(* Logix 5000 AddOnInstructionDefinition export B256_LtoE; software revision 30.00 *)

ADD_ON_INSTRUCTION D_SHR   (* revision 1.0, vendor Ken Fischer, NSWCPD, C512 *)
// DINT bit shift right of the 32-bit argument Inp_A by Inp_B bits with paddding by zeros on the right
// Revision note:
// Rev1.0: TBD - Initial Release
VAR_IN_OUT
   Inp_A : DINT; {required}   // 64-bit Integer to be right circular rotated
END_VAR
VAR_INPUT
   Inp_B : INT; {required}   // Number of bits to shift
END_VAR
VAR_IN_OUT
   Out : DINT; {required}   // Result
END_VAR
VAR
   BSR_Cntrl : CONTROL := (LEN := 32);
   ONS : BOOL;
   Source_Bit : BOOL;
   Wrk_InpA : DINT[2];
END_VAR

ROUTINE Logic   (* ladder *)
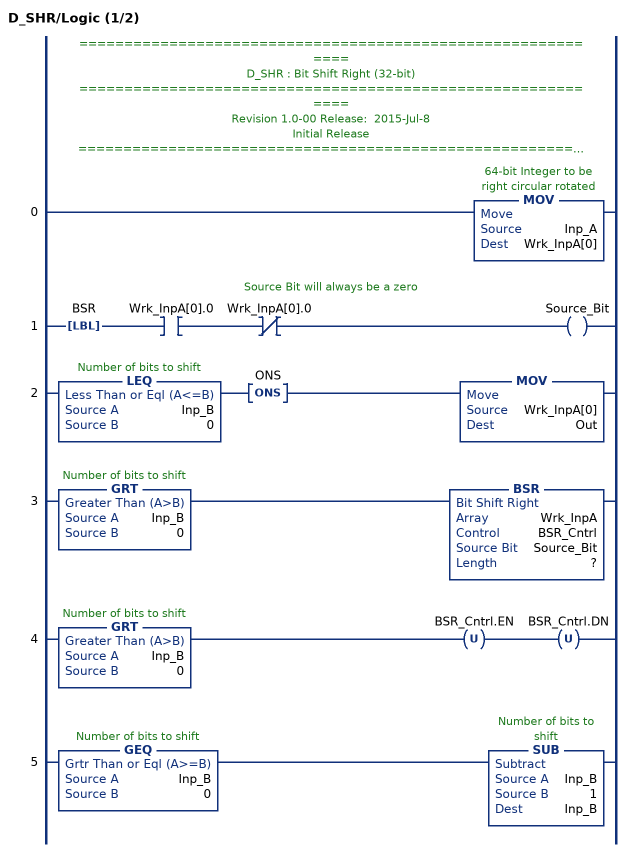
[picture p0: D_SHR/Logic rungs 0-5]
   // ============================================================
   // D_SHR : Bit Shift Right (32-bit)
   // ============================================================
   // Revision 1.0-00 Release:  2015-Jul-8
   // Initial Release
   // ============================================================
   // Performs a right bit shift of the 32-bit argument Inp_A by the
   // number of bits defined in the 16-bit argument Inp_B, with padding by zeros.
   0: MOV(Inp_A,Wrk_InpA[0]);
   // Source Bit will always be a zero
   1: LBL(BSR)XIC(Wrk_InpA[0].0)XIO(Wrk_InpA[0].0)OTE(Source_Bit);
   2: LEQ(Inp_B,0)ONS(ONS)MOV(Wrk_InpA[0],Out);
   3: GRT(Inp_B,0)BSR(Wrk_InpA,BSR_Cntrl,Source_Bit,?);
   4: GRT(Inp_B,0)OTU(BSR_Cntrl.EN)OTU(BSR_Cntrl.DN);
   5: GEQ(Inp_B,0)SUB(Inp_B,1,Inp_B);
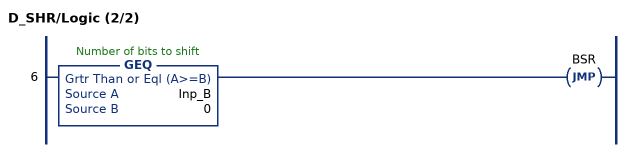
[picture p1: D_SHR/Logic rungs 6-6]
   6: GEQ(Inp_B,0)JMP(BSR);
END_ROUTINE
END_ADD_ON_INSTRUCTION

ADD_ON_INSTRUCTION B256_LtoE   (* revision 1.0 20170916, vendor Kenneth A. Fischer *)
// Convert 256-bit value using 4 64-bit pieces into 256-bit value using 32 8-bit pieces
// Revision note:
// Rev1.0: 20170916 - Initial Release
VAR_IN_OUT
   Inp_L : LINT[4]; {required}
   Out_E : DINT[32]; {required}
END_VAR
VAR
   i : INT;
   j : INT;
   Wrk_InpL : DINT[2];
   D_SHR : D_SHR;
   TEMP : DINT;
END_VAR

ROUTINE Logic   (* ladder *)
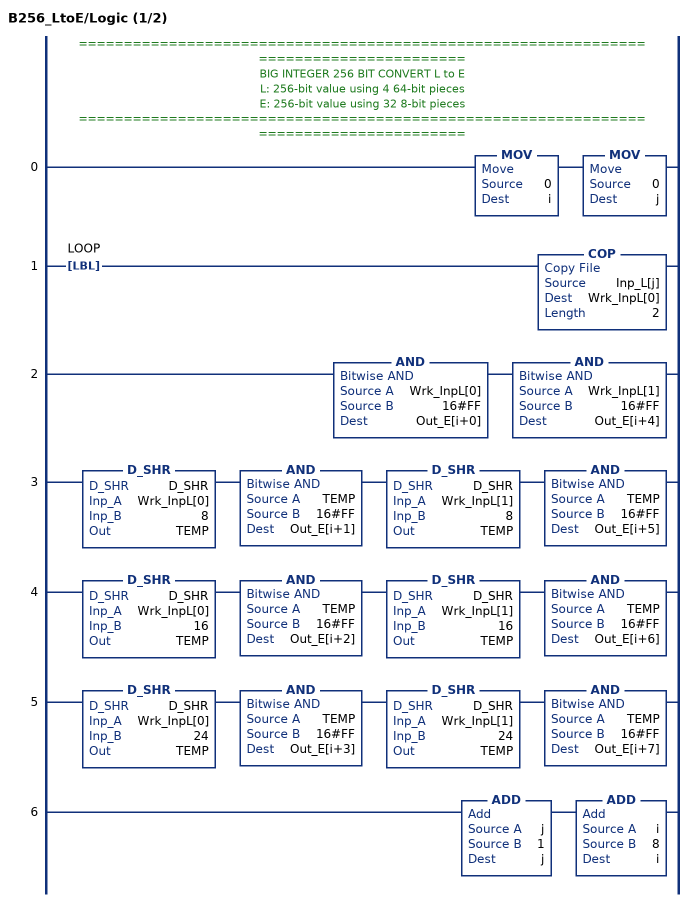
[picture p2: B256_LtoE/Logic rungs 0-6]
   // ======================================================================================
   // BIG INTEGER 256 BIT CONVERT L to E
   // L: 256-bit value using 4 64-bit pieces
   // E: 256-bit value using 32 8-bit pieces
   // ======================================================================================
   0: MOV(0,i)MOV(0,j);
   1: LBL(LOOP)COP(Inp_L[j],Wrk_InpL[0],2);
   2: AND(Wrk_InpL[0],16#FF,Out_E[i+0])AND(Wrk_InpL[1],16#FF,Out_E[i+4]);
   3: D_SHR(D_SHR,Wrk_InpL[0],8,TEMP)AND(TEMP,16#FF,Out_E[i+1])D_SHR(D_SHR,Wrk_InpL[1],8,TEMP)AND(TEMP,16#FF,Out_E[i+5]);
   4: D_SHR(D_SHR,Wrk_InpL[0],16,TEMP)AND(TEMP,16#FF,Out_E[i+2])D_SHR(D_SHR,Wrk_InpL[1],16,TEMP)AND(TEMP,16#FF,Out_E[i+6]);
   5: D_SHR(D_SHR,Wrk_InpL[0],24,TEMP)AND(TEMP,16#FF,Out_E[i+3])D_SHR(D_SHR,Wrk_InpL[1],24,TEMP)AND(TEMP,16#FF,Out_E[i+7]);
   6: ADD(j,1,j)ADD(i,8,i);
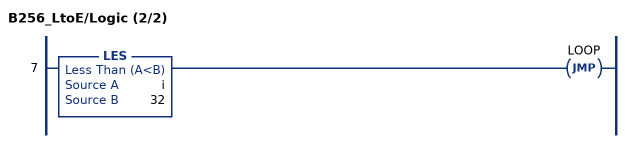
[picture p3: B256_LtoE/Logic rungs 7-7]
   7: LES(i,32)JMP(LOOP);
END_ROUTINE
END_ADD_ON_INSTRUCTION
